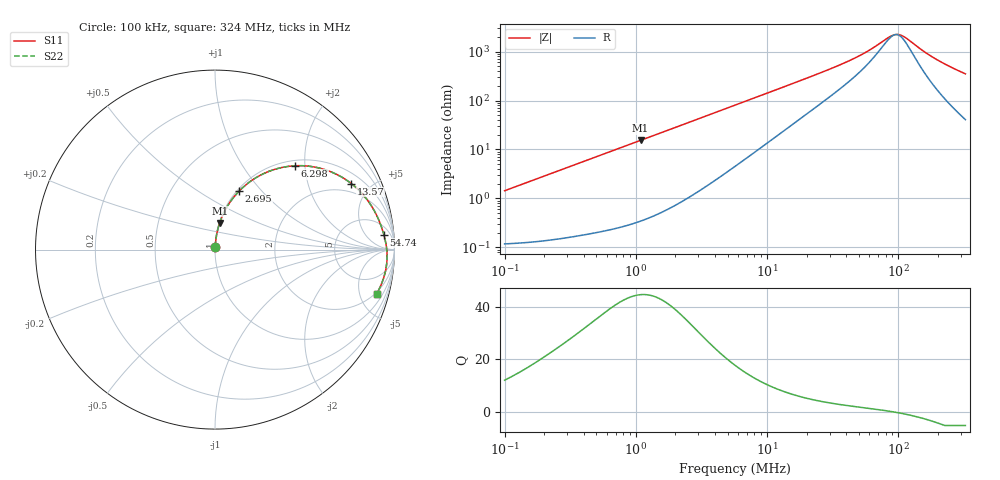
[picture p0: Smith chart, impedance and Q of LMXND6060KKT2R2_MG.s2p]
! LMXND6060KKT2R2_MG  S-PARAMETER MODEL  ( General Type )
! Model Generated by TAIYO YUDEN Corporation (http://www.ty-top.com)
! Version 1.0
! TAIYO YUDEN Control No. 191023NI43SB-FBB
! Copyright(c) 2019 TAIYO YUDEN CO.,LTD. All Rights Reserved.
! Product Description (link to TY-COMPAS)
! https://ds.yuden.co.jp/TYCOMPAS/or/detail?pn=LMXND6060KKT2R2MMG&u=M
! Products Name : Inductors
! Characteristics :
!  Inductance : 2.2 uH , SRF(min) : 56 MHz , DC Resistance(max) : 0.132 Ohm
!  Rated Current : Saturation :1900 mA , Temp Rise : 1700 mA
!  Case Size : 6.0 x 6.0 / 0.236 x 0.236 [mm/inch] , Thickness : 1 / 0.039 [mm/inch]
!  (Conditions: Temperature = 25 degC , DC Bias Current/Voltage = 0A / 0V)
! External Node Assignments :
!  1  o---GGG---o  2
! GND o---------o GND
! Frequency Range : 0.1MHz  -  324.04089MHz  [ 402 STEP ]
# MHz S RI R 50
! Freq[MHz].  S11 Real  S11 Imag  S21 Real  S21 Imag  S12 Real  S12 Imag  S22 Real  S22 Imag
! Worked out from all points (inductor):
!   401 points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, 100 kHz to 324 MHz, reference 50 ohm
!   read as one part in series: L = 2.28 uH near 104.1 kHz
!   highest Q = 44.6 at 1.085 MHz (marker M1), where L = 2.24 uH
!   self-resonance near 95.15 MHz
!   S11 on the Smith chart (normalised r, x): 100 kHz: 1.00, +0.03; 2.695 MHz: 1.02, +0.76; 6.298 MHz: 1.11, +1.77; 13.57 MHz: 1.49, +3.81; 54.74 MHz: 10, +16; 324 MHz: 1.81, -6.95
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0.1  0.00138 0.0143  0.9986 -0.0143  0.9986 -0.0143  0.00138 0.0143
0.38728  0.00476 0.0546  0.9952 -0.0546  0.9952 -0.0546  0.00476 0.0546
0.66833  0.0111 0.0932  0.9889 -0.0932  0.9889 -0.0932  0.0111 0.0932
1.085493  0.0261 0.1486  0.9739 -0.1486  0.9739 -0.1486  0.0261 0.1486
1.499861  0.047 0.2005  0.953 -0.2005  0.953 -0.2005  0.047 0.2005
2.695066  0.1335 0.3252  0.8665 -0.3252  0.8665 -0.3252  0.1335 0.3252
3.877452  0.2388 0.4067  0.7612 -0.4067  0.7612 -0.4067  0.2388 0.4067
5.692459  0.3973 0.4621  0.6027 -0.4621  0.6027 -0.4621  0.3973 0.4621
6.297706  0.4443 0.467  0.5557 -0.467  0.5557 -0.467  0.4443 0.467
8.879385  0.6025 0.4486  0.3975 -0.4486  0.3975 -0.4486  0.6025 0.4486
13.57342  0.7597 0.3677  0.2403 -0.3677  0.2403 -0.3677  0.7597 0.3677
22.04577  0.8658 0.2525  0.1342 -0.2525  0.1342 -0.2525  0.8658 0.2525
37.2833  0.92 0.1463  0.08 -0.1463  0.08 -0.1463  0.92 0.1463
54.73535  0.9407 0.0837  0.0593 -0.0837  0.0593 -0.0837  0.9407 0.0837
85.37896  0.9549 0.0167  0.0451 -0.0167  0.0451 -0.0167  0.9549 0.0167
96.38509  0.9571 -0.00202  0.0429 0.00202  0.0429 0.00202  0.9571 -0.00202
106.6332  0.9583 -0.0181  0.0417 0.0181  0.0417 0.0181  0.9583 -0.0181
117.9709  0.9588 -0.0347  0.0412 0.0347  0.0412 0.0347  0.9588 -0.0347
156.5474  0.9559 -0.0848  0.0441 0.0848  0.0441 0.0848  0.9559 -0.0848
187.7735  0.9498 -0.1205  0.0502 0.1205  0.0502 0.1205  0.9498 -0.1205
249.1755  0.9311 -0.1825  0.0689 0.1825  0.0689 0.1825  0.9311 -0.1825
324.0409  0.9 -0.2472  0.1 0.2472  0.1 0.2472  0.9 -0.2472
